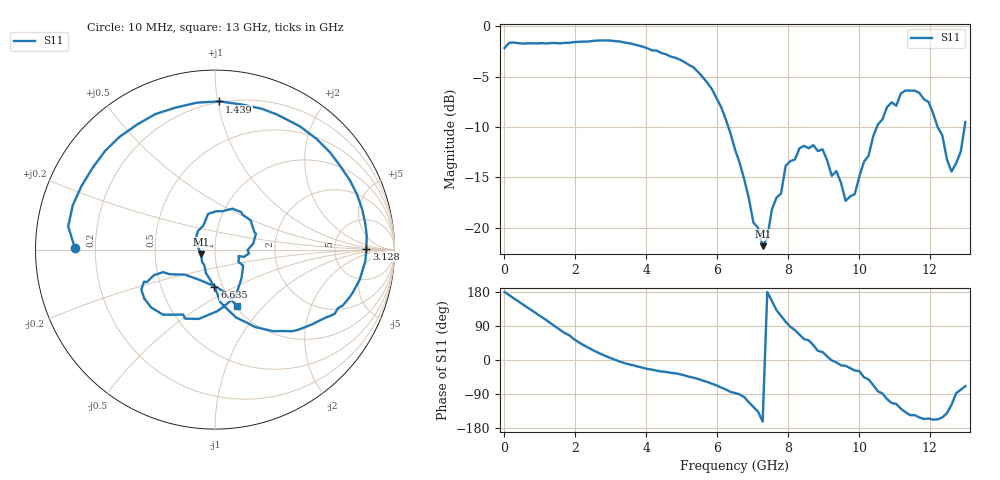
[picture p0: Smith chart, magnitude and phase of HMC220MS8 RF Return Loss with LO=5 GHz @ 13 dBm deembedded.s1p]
!Hittite Microwave Corporation
!12 Elizabeth Drive
!Chelmsford, MA 01824
!Tel: 978-250-3343
!Fax: 978-250-3373
!Device: HMC220MS8, 5-12 GHz, GaAS MMIC SMT Double-Balanced Mixer in 8-lead MSOP package
!Misc: RF Return Loss, LO = 5 GHz @ 13dBm, Room
# MHZ S MA R 50
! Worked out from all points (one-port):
!   101 points, 10 MHz to 13 GHz, reference 50 ohm
!   lowest |S11| = -21.8 dB at 7.284 GHz (marker M1), VSWR 1.18, Z = 42.8 - j2.1 ohm
!   |S11| at or under -10 dB: 6.317 GHz to 10.5 GHz (4.187 GHz wide, 49.8 % of centre); 12.22 GHz to 12.98 GHz (760.4 MHz wide, 6.04 % of centre)
!   S11 on the Smith chart (normalised r, x): 10 MHz: 0.12, +0.00; 1.439 GHz: 0.19, +1.01; 3.128 GHz: 12, +0; 6.635 GHz: 0.91, -0.40; 13 GHz: 1.02, -0.72
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10  0.78 179.5
269.8  0.83 162.7
659.5  0.823 138.0
1049.2  0.825 113.8
1438.9  0.826 88.3
1698.7  0.827 71.6
2088.4  0.837 47.4
2478.1  0.845 27.0
3127.6  0.843 0.4
3257.5  0.84 -4.2
4036.9  0.777 -23.6
4946.2  0.684 -37.4
5855.5  0.487 -62.5
6505  0.245 -87.1
6634.9  0.21 -90.9
7284.4  0.081 -162.4
7933.9  0.203 100.9
8193.7  0.218 78.9
8973.1  0.245 21.2
9622.6  0.136 -15.3
9752.5  0.143 -21.6
10402  0.285 -66.3
10791.7  0.397 -103.3
11441.2  0.479 -145.6
11960.8  0.421 -154.5
12610.3  0.19 -117.9
12870.1  0.239 -78.5
13000  0.335 -68.7
